(* Logix 5000 AddOnInstructionDefinition export NTEC_MAH; software revision ? *)

TYPE NTEC_Axis :   // NTEC Axis:
STRUCT
   StatDriveCommsOK : BOOL;   // Drive is communicating over ENET IP
   StatServoActionStatus : BOOL;   // Motion is enabled and holding position under power.
   StatDriveWarning : BOOL;   // Drive has a Warning
   StatDriveFault : BOOL;   // Drive is Faulted
   StatMotion_AtTarget : BOOL;   // Motion Target Reached
   StatMotion_FollowingError : BOOL;   // Following Error Fault
   StatMotion_LimitExceeded : BOOL;   // Speed or Position Limit Exceeded
   StatMotion_Halt : BOOL;   // Motor is in Halt, still powered on
   StatQuckStop : BOOL;   // Motor is powered off in Quick Stop
   StatMotion_Homed : BOOL;   // Motion Coordinate System Homed
   StatNewCmdToggle : BOOL;   // Bit toggles after new command accepted
   StatCommandError : BOOL;   // Last Command has an Error
   StatCommandErrorCode : DINT;   // Command Error Code
   StatDriveFaultCode : DINT;   // Drive Fault Code
   StatDriveWarningCode : DINT;   // Drive Warning Code
   StatResettingFault : BOOL;   // In fault reset sequence
   StatReadResponse : DINT;   // Response from a Read CMD
   CMD_IP : BOOL;   // Command is In Process
   CMD_DN : BOOL;   // Command is Done
   CMD_ERR : BOOL;   // Command Error during Comms send to Drive
   PDI_CMD : NTEC_PDI_CMD;   // Commands from AOIs
   PDI_Status : NTEC_PDI_Status;   // Status from Drive out to AOIs
   DriveLimits : NTEC_LimitsInDrive;   // Limits read from Drive
END_STRUCT
END_TYPE

TYPE NTEC_LimitsInDrive :   // These are the limits read from the Drive
STRUCT
   PositionLimitMin : DINT;   // Minimum Allowed Position Target (607Bh:1)
   PositionLimitMax : DINT;   // Maximum Allowed Position Target (607Bh:2)
   SoftPositionLimitMin : DINT;   // Minimum Allowed Position (607Dh:1)
   SoftPositionLimitMax : DINT;   // Minimum Allowed Position (607Dh:2)
   VelocityLimitMin : DINT;   // Maximum Allowed Velocity Target negative direction
   VelocityLimitMax : DINT;   // Maximum Allowed Velocity Target positive direction (607Fh)
   MotorSpeedMin : DINT;   // Maximum motor speed in negative direction
   MotorSpeedMax : DINT;   // Maximum motor speed setting in positive direction (6080h)
   AccelLimitMax : DINT;   // Maximum Allowed Accel Target (60C5h)
   DecelLimitMax : DINT;   // Maximum Allowed Decel Target (60C6h)
   PositionWindowNeg : DINT;   // Position Window - negative direction for At Target (6067h)
   PositionWindowPos : DINT;   // Position Window -positive direction for At Target (+/- this value) (6067h)
   VelocityWindowNeg : DINT;   // Velocity Window - negative side for At Target (+/- this value) (606Dh)
   VelocityWindowPos : DINT;   // Velocity Window - positive side for At Target (+/- this value) (606Dh)
   TorqueMaxNegDir : DINT;   // Maximum Torque Target negative direction (0.1% of motor rated current 2031h) (6072h)
   TorqueMaxPosDir : DINT;   // Maximum Torque Target positive direction (0.1% of motor rated current 2031h) (6072h)
   CurrentMaxNegDir : DINT;   // Maximum Current Target negative direction (in 0.1% of rated setting 2031h) (6073h)
   CurrentMaxPosDir : DINT;   // Maximum Current Target positive direction (in 0.1% of rated setting 2031h) (6073h)
END_STRUCT
END_TYPE

TYPE NTEC_PDI_CMD :   // PDI Command Bytes
STRUCT
   SetValue1 : DINT;
   SetValue2 : INT;
   SetValue3 : SINT;
   CMD : SINT;
   DigitalOutputs : DINT;
   NanoJ_Input1 : DINT;
   Trig : BOOL;   // Trigger the Command
   Halt : BOOL;   // Command a HALT
   QuickStop : BOOL;   // Command a QuickStop
END_STRUCT
END_TYPE

TYPE NTEC_PDI_Status :   // PDI Status Bytes
STRUCT
   Status : INT;
   ErrorCode : INT;
   ReturnValue : DINT;
   PositionActualValue : DINT;
   VelocityActualValue : DINT;
   DigitalInputs : DINT;
   TorqueActualValue : INT;
   AnalogInput1 : INT;
   FollowingError : DINT;
   NanoJ_Output1 : DINT;
END_STRUCT
END_TYPE

ADD_ON_INSTRUCTION NTEC_MAH   (* revision 1.6, vendor Third Coast Automation, Nashville, TN, ExecutePrescan, ExecuteEnableInFalse *)
// Motion Axis Home (MAH)
// Homes the servo axis position to a specified value at a specified location.  User to enter the Home Type (1=Immediate, 2=Sensor, 3=Block)  and if applicable, the Homing Method (matched up to values set in Drive using Plug & Drive software).
// All input parameters are entered into the AOI in whole numbers, in the units as setup and scaled in the Drive.
// Revision note:
// Release Aug 27, 2024, update CPS instructions LEN
// Help:
// AOI written by:
// Tim Cochran
// Third Coast Automation
// Nashville, TN
// Home Instruction for Nanotec Drives.
// Position = Coordinate position set after home is complete.
// HomeType 1=Immediate, 2=Sensor, 3=Block (HardStop).
// Home Method is from the Technical Manual, applicable to Sensor or Block homing. Best to setup and test the home method number/parameters and test using Plug & Drive software for reliable results.
// MAH ERR_Codes:
// 2: Input parameter range error – review and fix input parameters.
// 3: Command Error response from the Drive after command sent.
// 10: Communications Failed to Drive.
// 11: Drive Fault during this AOIs command sequence.
// 12: Quick Stop triggered by software outside of this AOI.
// 13: Command Error response from the Drive.
// 14: Enable input changed to False during sequence due to Drive Fault or Offline.
VAR_IN_OUT
   NTEC_Axis : NTEC_Axis; {required}   // NTEC Axis Tag
END_VAR
VAR_INPUT
   Position : DINT; {required}   // Position value for home location
   HomeType : DINT; {required}   // 1=Immediate 2=Sensor 3=Block
   HomeMethod : DINT; {required}   // Nanotec Drive Homing Method, 1 to 34, for Sensor/Block homing
END_VAR
VAR_OUTPUT
   EN : BOOL; {access Read Only, visible}   // Enabled
   IP : BOOL; {visible}   // In Process
   DN : BOOL; {visible}   // Successfully Done
   ERR : BOOL; {visible}   // Instruction Error
   ERR_Code : DINT; {access Read Only, visible}   // Instruction Error Code
END_VAR
VAR
   State : DINT; {access None}
   Enable : BOOL; {access None}
   local_HomeType : DINT; {access None}
   local_Position : DINT; {access None}
   local_HomeMethod : DINT; {access None}
   InputRangesOK : BOOL; {access None}
   tmr_VerifyHomedInput : TIMER := (PRE := 200); {access None}
   ServoActionWatchdog : TIMER := (PRE := 1000); {access None}
END_VAR

ROUTINE EnableInFalse   (* ladder *)
// Enable In False Routine
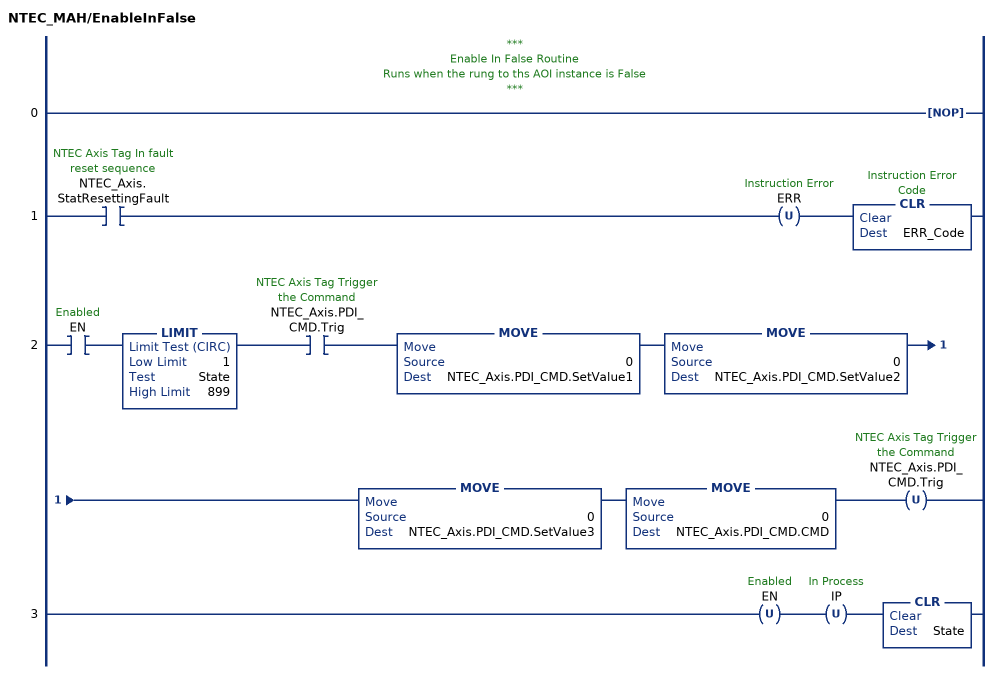
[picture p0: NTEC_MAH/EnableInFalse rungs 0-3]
   // ***
   // Enable In False Routine
   // Runs when the rung to ths AOI instance is False
   // ***
   0: NOP();
   1: XIC(NTEC_Axis.StatResettingFault)OTU(ERR)CLR(ERR_Code);
   2: XIC(EN)LIMIT(1,State,899)XIC(NTEC_Axis.PDI_CMD.Trig)MOVE(0,NTEC_Axis.PDI_CMD.SetValue1)MOVE(0,NTEC_Axis.PDI_CMD.SetValue2)MOVE(0,NTEC_Axis.PDI_CMD.SetValue3)MOVE(0,NTEC_Axis.PDI_CMD.CMD)OTU(NTEC_Axis.PDI_CMD.Trig);
   3: OTU(EN)OTU(IP)CLR(State);
END_ROUTINE

ROUTINE Logic   (* ladder *)
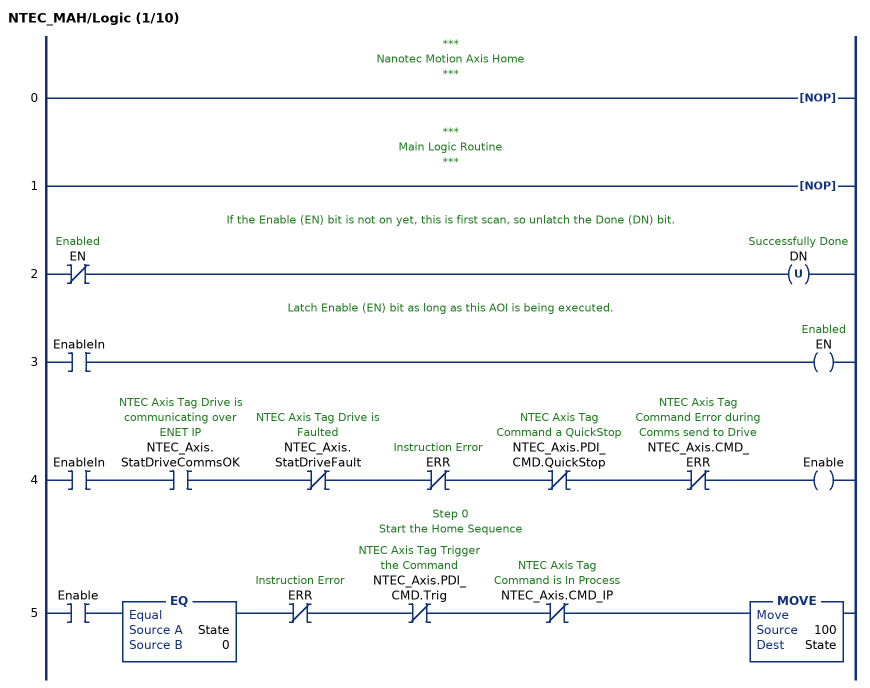
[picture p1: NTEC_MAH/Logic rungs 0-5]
   // ***
   // Nanotec Motion Axis Home
   // ***
   0: NOP();
   // ***
   // Main Logic Routine
   // ***
   1: NOP();
   // If the Enable (EN) bit is not on yet, this is first scan, so unlatch the Done (DN) bit.
   2: XIO(EN)OTU(DN);
   // Latch Enable (EN) bit as long as this AOI is being executed.
   3: XIC(EnableIn)OTE(EN);
   4: XIC(EnableIn)XIC(NTEC_Axis.StatDriveCommsOK)XIO(NTEC_Axis.StatDriveFault)XIO(ERR)XIO(NTEC_Axis.PDI_CMD.QuickStop)XIO(NTEC_Axis.CMD_ERR)OTE(Enable);
   // Step 0
   // Start the Home Sequence
   5: XIC(Enable)EQ(State,0)XIO(ERR)XIO(NTEC_Axis.PDI_CMD.Trig)XIO(NTEC_Axis.CMD_IP)MOVE(100,State);
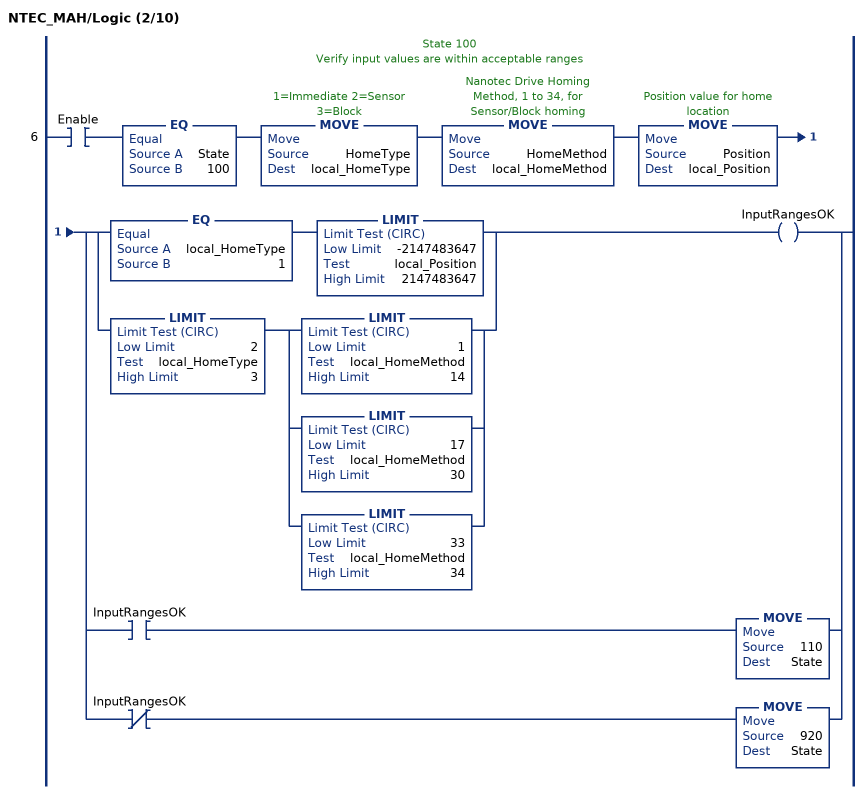
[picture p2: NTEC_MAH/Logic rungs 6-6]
   // State 100
   // Verify input values are within acceptable ranges
   6: XIC(Enable)EQ(State,100)MOVE(HomeType,local_HomeType)MOVE(HomeMethod,local_HomeMethod)MOVE(Position,local_Position)[[EQ(local_HomeType,1) LIMIT(-2147483647,local_Position,2147483647) ,LIMIT(2,local_HomeType,3) [LIMIT(1,local_HomeMethod,14) ,LIMIT(17,local_HomeMethod,30) ,LIMIT(33,local_HomeMethod,34) ] ] OTE(InputRangesOK) ,XIC(InputRangesOK) MOVE(110,State) ,XIO(InputRangesOK) MOVE(920,State) ];
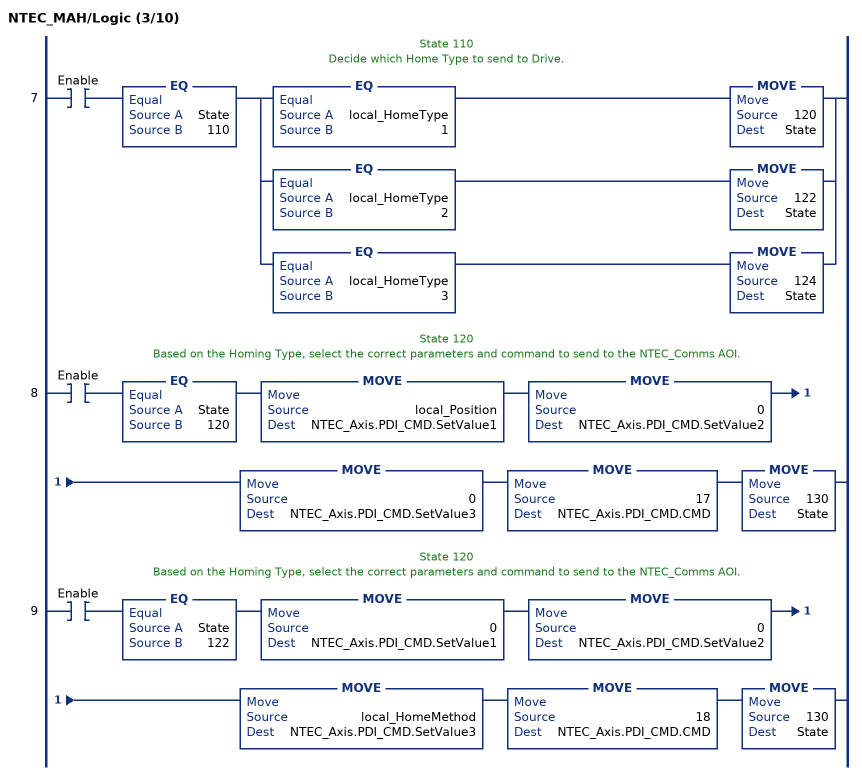
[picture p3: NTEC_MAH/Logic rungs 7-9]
   // State 110
   // Decide which Home Type to send to Drive.
   7: XIC(Enable)EQ(State,110)[EQ(local_HomeType,1) MOVE(120,State) ,EQ(local_HomeType,2) MOVE(122,State) ,EQ(local_HomeType,3) MOVE(124,State) ];
   // State 120
   // Based on the Homing Type, select the correct parameters and command to send to the NTEC_Comms AOI.
   8: XIC(Enable)EQ(State,120)MOVE(local_Position,NTEC_Axis.PDI_CMD.SetValue1)MOVE(0,NTEC_Axis.PDI_CMD.SetValue2)MOVE(0,NTEC_Axis.PDI_CMD.SetValue3)MOVE(17,NTEC_Axis.PDI_CMD.CMD)MOVE(130,State);
   // State 120
   // Based on the Homing Type, select the correct parameters and command to send to the NTEC_Comms AOI.
   9: XIC(Enable)EQ(State,122)MOVE(0,NTEC_Axis.PDI_CMD.SetValue1)MOVE(0,NTEC_Axis.PDI_CMD.SetValue2)MOVE(local_HomeMethod,NTEC_Axis.PDI_CMD.SetValue3)MOVE(18,NTEC_Axis.PDI_CMD.CMD)MOVE(130,State);
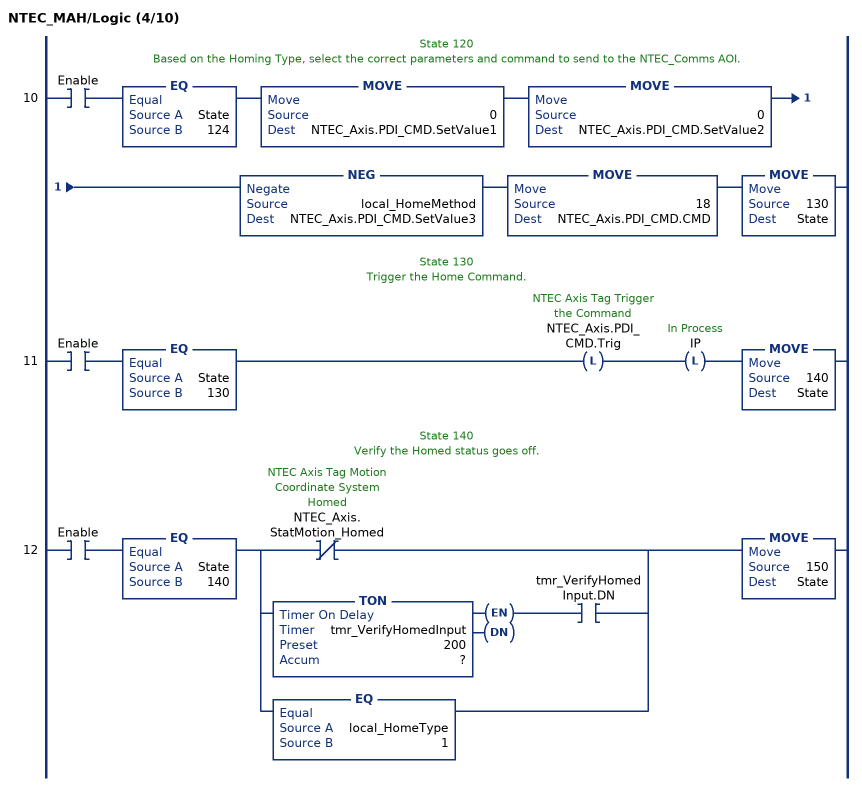
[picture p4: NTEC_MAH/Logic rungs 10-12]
   // State 120
   // Based on the Homing Type, select the correct parameters and command to send to the NTEC_Comms AOI.
   10: XIC(Enable)EQ(State,124)MOVE(0,NTEC_Axis.PDI_CMD.SetValue1)MOVE(0,NTEC_Axis.PDI_CMD.SetValue2)NEG(local_HomeMethod,NTEC_Axis.PDI_CMD.SetValue3)MOVE(18,NTEC_Axis.PDI_CMD.CMD)MOVE(130,State);
   // State 130
   // Trigger the Home Command.
   11: XIC(Enable)EQ(State,130)OTL(NTEC_Axis.PDI_CMD.Trig)OTL(IP)MOVE(140,State);
   // State 140
   // Verify the Homed status goes off.
   12: XIC(Enable)EQ(State,140)[XIO(NTEC_Axis.StatMotion_Homed) ,TON(tmr_VerifyHomedInput,?,?) XIC(tmr_VerifyHomedInput.DN) ,EQ(local_HomeType,1) ]MOVE(150,State);
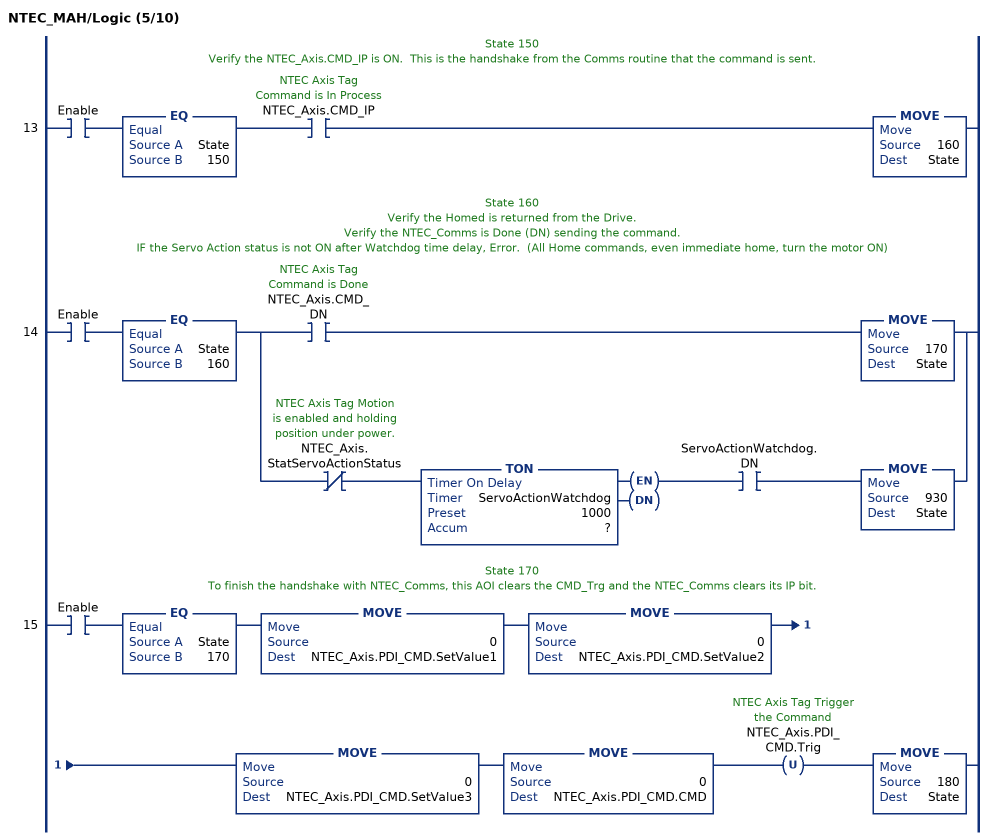
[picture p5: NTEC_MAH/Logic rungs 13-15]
   // State 150
   // Verify the NTEC_Axis.CMD_IP is ON.  This is the handshake from the Comms routine that the command is sent.
   13: XIC(Enable)EQ(State,150)XIC(NTEC_Axis.CMD_IP)MOVE(160,State);
   // State 160
   // Verify the Homed is returned from the Drive.
   // Verify the NTEC_Comms is Done (DN) sending the command.
   // IF the Servo Action status is not ON after Watchdog time delay, Error.  (All Home commands, even immediate home, turn the motor ON)
   14: XIC(Enable)EQ(State,160)[XIC(NTEC_Axis.CMD_DN) MOVE(170,State) ,XIO(NTEC_Axis.StatServoActionStatus) TON(ServoActionWatchdog,?,?) XIC(ServoActionWatchdog.DN) MOVE(930,State) ];
   // State 170
   // To finish the handshake with NTEC_Comms, this AOI clears the CMD_Trg and the NTEC_Comms clears its IP bit.
   15: XIC(Enable)EQ(State,170)MOVE(0,NTEC_Axis.PDI_CMD.SetValue1)MOVE(0,NTEC_Axis.PDI_CMD.SetValue2)MOVE(0,NTEC_Axis.PDI_CMD.SetValue3)MOVE(0,NTEC_Axis.PDI_CMD.CMD)OTU(NTEC_Axis.PDI_CMD.Trig)MOVE(180,State);
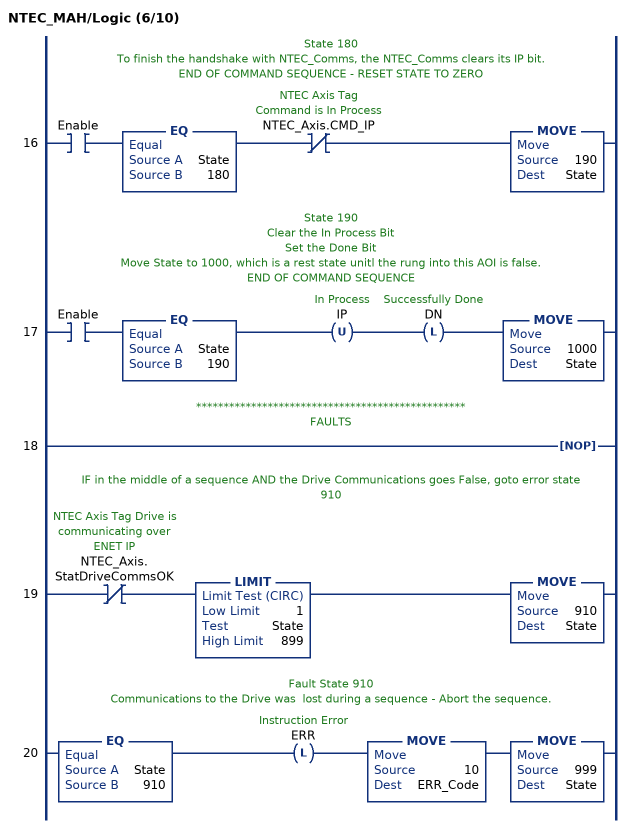
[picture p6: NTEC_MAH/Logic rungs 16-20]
   // State 180
   // To finish the handshake with NTEC_Comms, the NTEC_Comms clears its IP bit.
   // END OF COMMAND SEQUENCE - RESET STATE TO ZERO
   16: XIC(Enable)EQ(State,180)XIO(NTEC_Axis.CMD_IP)MOVE(190,State);
   // State 190
   // Clear the In Process Bit
   // Set the Done Bit
   // Move State to 1000, which is a rest state unitl the rung into this AOI is false.
   // END OF COMMAND SEQUENCE
   17: XIC(Enable)EQ(State,190)OTU(IP)OTL(DN)MOVE(1000,State);
   // *************************************************
   // FAULTS
   18: NOP();
   // IF in the middle of a sequence AND the Drive Communications goes False, goto error state 910
   19: XIO(NTEC_Axis.StatDriveCommsOK)LIMIT(1,State,899)MOVE(910,State);
   // Fault State 910
   // Communications to the Drive was  lost during a sequence - Abort the sequence.
   20: EQ(State,910)OTL(ERR)MOVE(10,ERR_Code)MOVE(999,State);
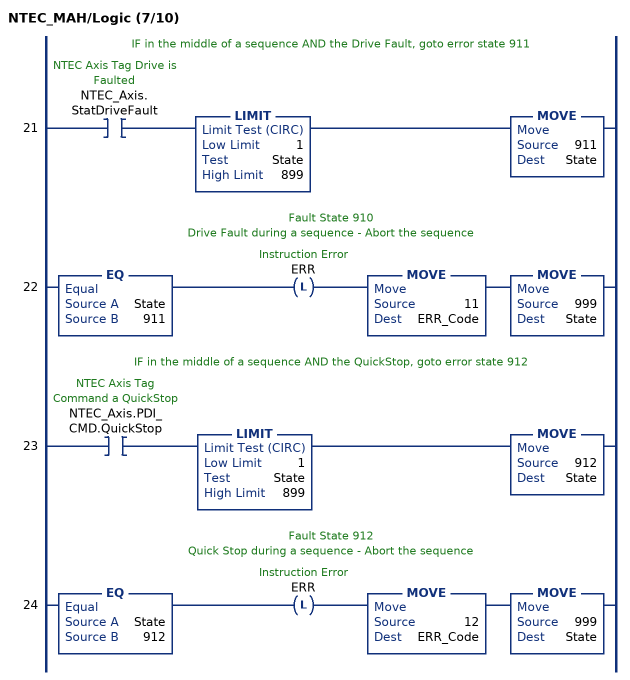
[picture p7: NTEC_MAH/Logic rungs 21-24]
   // IF in the middle of a sequence AND the Drive Fault, goto error state 911
   21: XIC(NTEC_Axis.StatDriveFault)LIMIT(1,State,899)MOVE(911,State);
   // Fault State 910
   // Drive Fault during a sequence - Abort the sequence
   22: EQ(State,911)OTL(ERR)MOVE(11,ERR_Code)MOVE(999,State);
   // IF in the middle of a sequence AND the QuickStop, goto error state 912
   23: XIC(NTEC_Axis.PDI_CMD.QuickStop)LIMIT(1,State,899)MOVE(912,State);
   // Fault State 912
   // Quick Stop during a sequence - Abort the sequence
   24: EQ(State,912)OTL(ERR)MOVE(12,ERR_Code)MOVE(999,State);
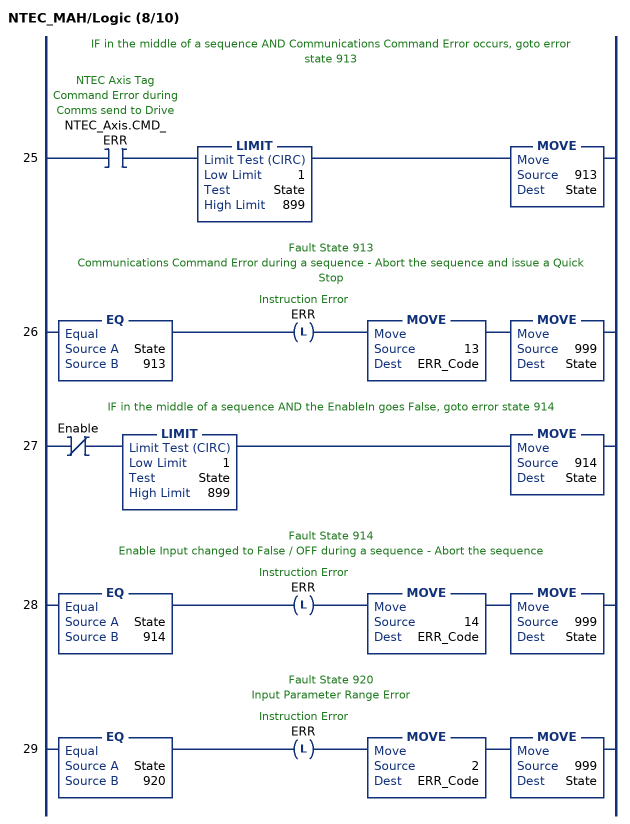
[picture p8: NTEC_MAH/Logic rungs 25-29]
   // IF in the middle of a sequence AND Communications Command Error occurs, goto error state 913
   25: XIC(NTEC_Axis.CMD_ERR)LIMIT(1,State,899)MOVE(913,State);
   // Fault State 913
   // Communications Command Error during a sequence - Abort the sequence and issue a Quick Stop
   26: EQ(State,913)OTL(ERR)MOVE(13,ERR_Code)MOVE(999,State);
   // IF in the middle of a sequence AND the EnableIn goes False, goto error state 914
   27: XIO(Enable)LIMIT(1,State,899)MOVE(914,State);
   // Fault State 914
   // Enable Input changed to False / OFF during a sequence - Abort the sequence
   28: EQ(State,914)OTL(ERR)MOVE(14,ERR_Code)MOVE(999,State);
   // Fault State 920
   // Input Parameter Range Error
   29: EQ(State,920)OTL(ERR)MOVE(2,ERR_Code)MOVE(999,State);
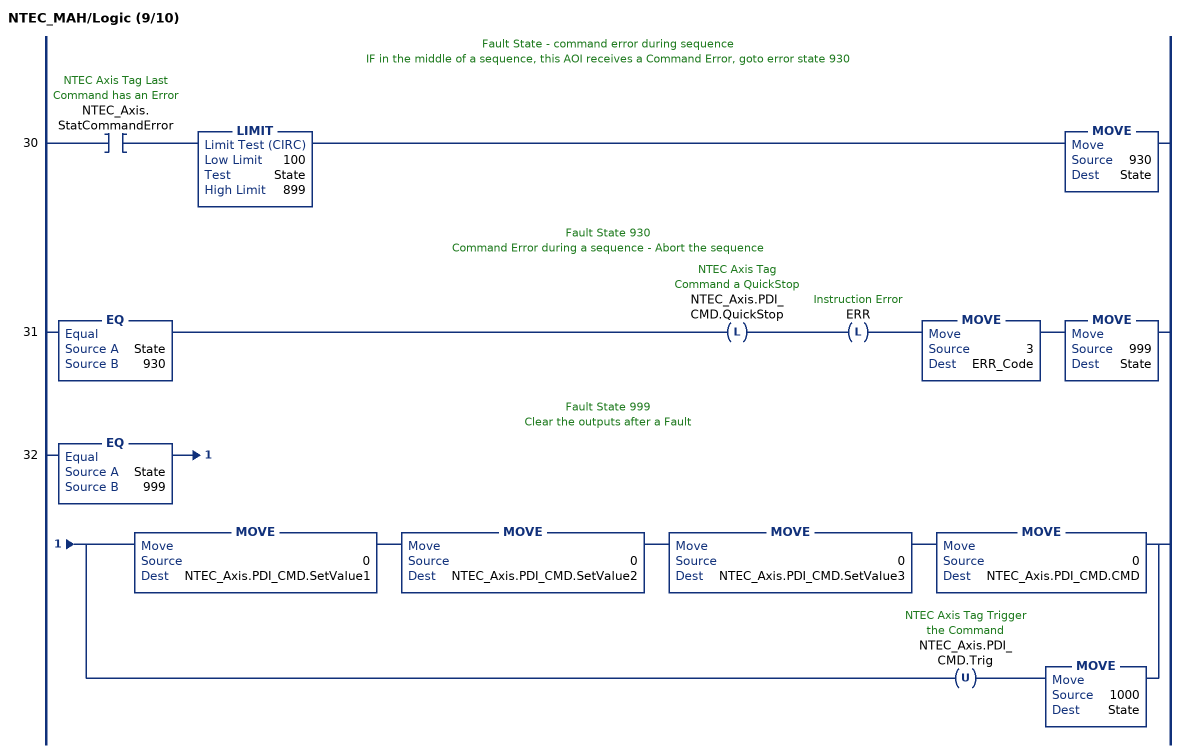
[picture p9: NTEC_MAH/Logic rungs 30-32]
   // Fault State - command error during sequence
   // IF in the middle of a sequence, this AOI receives a Command Error, goto error state 930
   30: XIC(NTEC_Axis.StatCommandError)LIMIT(100,State,899)MOVE(930,State);
   // Fault State 930
   // Command Error during a sequence - Abort the sequence
   31: EQ(State,930)OTL(NTEC_Axis.PDI_CMD.QuickStop)OTL(ERR)MOVE(3,ERR_Code)MOVE(999,State);
   // Fault State 999
   // Clear the outputs after a Fault
   32: EQ(State,999)[MOVE(0,NTEC_Axis.PDI_CMD.SetValue1) MOVE(0,NTEC_Axis.PDI_CMD.SetValue2) MOVE(0,NTEC_Axis.PDI_CMD.SetValue3) MOVE(0,NTEC_Axis.PDI_CMD.CMD) ,OTU(NTEC_Axis.PDI_CMD.Trig) MOVE(1000,State) ];
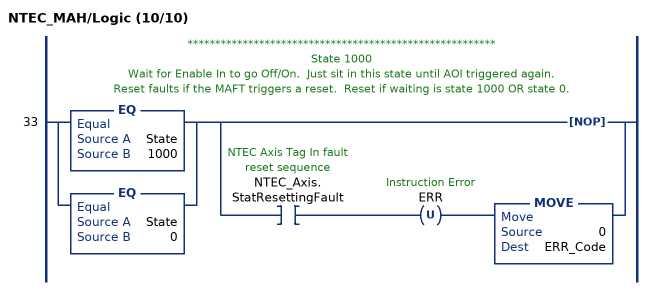
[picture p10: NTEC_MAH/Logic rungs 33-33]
   // ********************************************************
   // State 1000
   // Wait for Enable In to go Off/On.  Just sit in this state until AOI triggered again.
   // Reset faults if the MAFT triggers a reset.  Reset if waiting is state 1000 OR state 0.
   33: [EQ(State,1000) ,EQ(State,0) ][NOP() ,XIC(NTEC_Axis.StatResettingFault) OTU(ERR) MOVE(0,ERR_Code) ];
END_ROUTINE

ROUTINE Postscan   (* ladder *)
// Home Post-Scan Routine
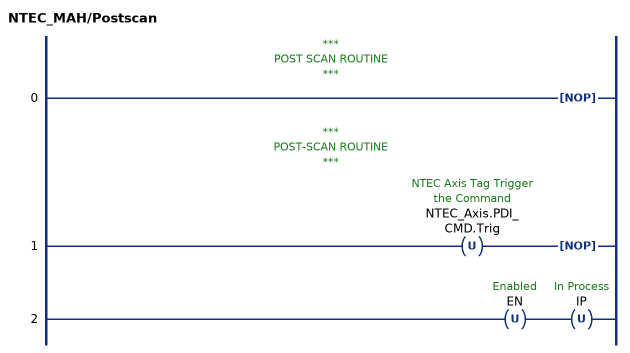
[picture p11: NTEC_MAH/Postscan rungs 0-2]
   // ***
   // POST SCAN ROUTINE
   // ***
   0: NOP();
   // ***
   // POST-SCAN ROUTINE
   // ***
   1: OTU(NTEC_Axis.PDI_CMD.Trig)NOP();
   2: OTU(EN)OTU(IP);
END_ROUTINE

ROUTINE Prescan   (* ladder *)
// Home Pre-Scan Routine
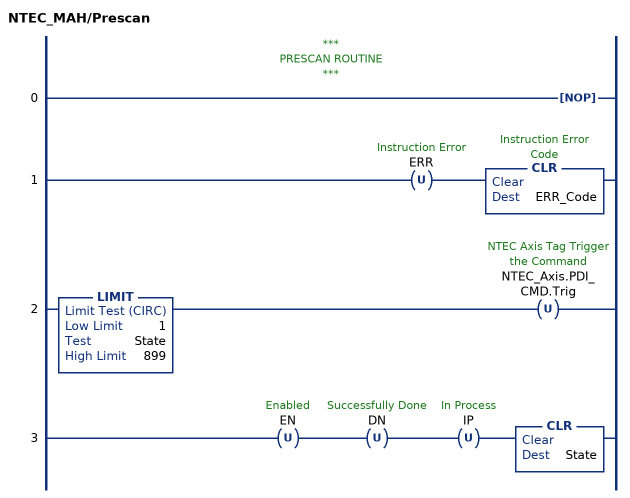
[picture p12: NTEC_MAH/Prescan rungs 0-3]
   // ***
   // PRESCAN ROUTINE
   // ***
   0: NOP();
   1: OTU(ERR)CLR(ERR_Code);
   2: LIMIT(1,State,899)OTU(NTEC_Axis.PDI_CMD.Trig);
   3: OTU(EN)OTU(DN)OTU(IP)CLR(State);
END_ROUTINE
END_ADD_ON_INSTRUCTION
